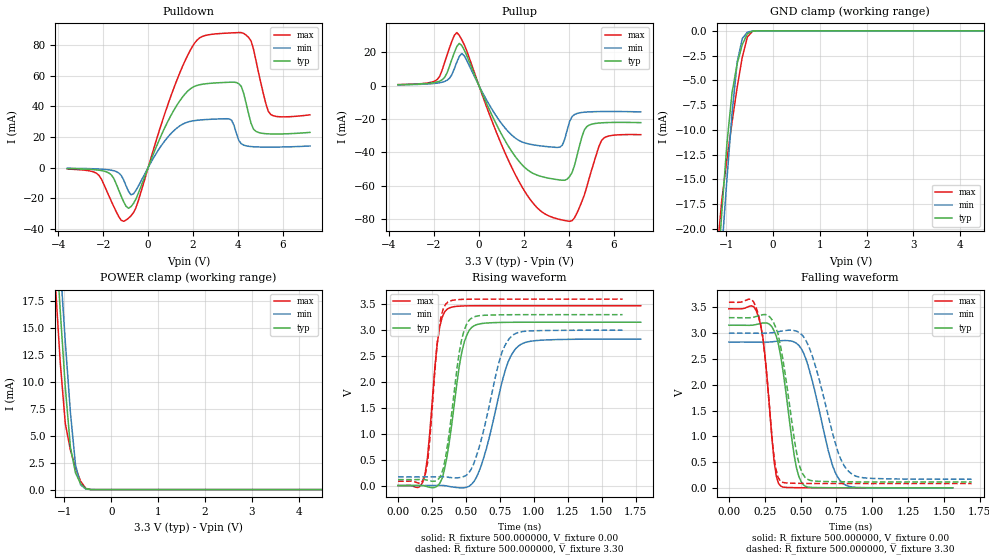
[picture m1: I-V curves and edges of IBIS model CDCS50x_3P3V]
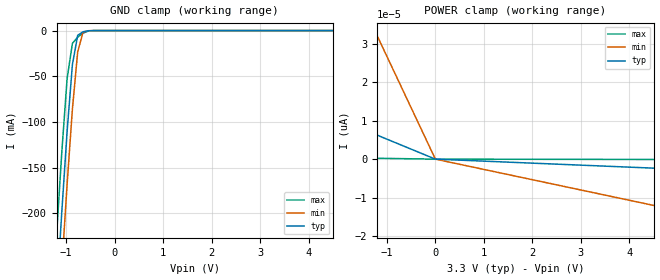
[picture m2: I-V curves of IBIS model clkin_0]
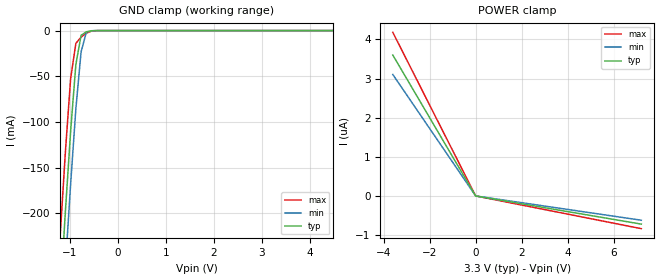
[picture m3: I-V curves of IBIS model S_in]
| TEXAS INSTRUMENTS INCORPORATED
| ASC / HSDC / CTS
| IBIS Model of CDCS504
| This file contains package information for the following:
| TSSOP-PW-8 package as [Component] CDCS504
| This device can be powered at the following Vccs:
| 3.3 volt
[IBIS Ver]   4.1
[Comment char]  |_char
[File Name]   cdcs504-q1.ibs
[File Rev]   1.0 | Simulation results only, no lab measurements
[Date]   April 27, 2017
[Source]   Model built from spectre simulations at:
   Texas Instruments Incorporated.
   Analog-eLab, HPA
   12500 TI Blvd
   Dallas, TX -75243
   For Support e-mail: webench_ibis_modeling@list.ti.com
[Notes]   Revision History
   Rev 1.0: 04/27/2017
[Disclaimer]  This model is designed as an aid for customers of Texas Instruments
 TI and its licensors and suppliers make no warranties, either expressed
 or implied, with respect to this  model, including the warranties of
 merchantability or fitness for a particular purpose.
 The model is provided solely on an "as is" basis. The entire risk as to
 its quality and performance is with the customer.
[Copyright] (C)Copyright 2017 Texas Instruments Incorporated.
   All rights reserved.
| Component TSSOP-PW-8 CDCS504
[Component]   CDCS504
[Manufacturer]   Texas Instruments, Inc.
[Package]
|   typ   min   max
R_pkg   0.747650e-01   0.368800e-01   1.126500e-01
L_pkg   1.018090e-09   0.602690e-09   1.433490e-09
C_pkg   1.006650e-13   6.656000e-14   1.347700e-13
[PIN]   signal_name   model_name   R_pin   L_pin   C_pin
1   IN   clkin_0   0.10191   1.26699e-09   0.08538e-12
2   GND   GND   0.10409   1.29915e-09   0.09128e-12
3   GND   POWER   0.05513   1.03439e-09   0.13141e-12
4   GND   POWER   0.08703   1.05334e-09   0.08277e-12
5   FS   S_in   0.03787   0.62719e-09   0.09930e-12
6   OUT   CDCS50x_3P3V   0.03688   0.60269e-09   0.09486e-12
7   OE   S_in   0.07828   0.93283e-09   0.06792e-12
8   VDD   POWER   0.07909   0.94459e-09   0.06676e-12
| Models and submodels in the file (3): CDCS50x_3P3V (Output), clkin_0 (Input), S_in (Input)
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[Model] CDCS50x_3P3V
|   Testbench Schematic CDCE949_3P3V model: Output
Model_type Output
Vmeas  =   1.50V
Cref   =   10.00pF
Rref   =   0
Vref   =   1.50V
| Variable   Typ   Min   Max
C_comp   1.113321e-12   1.105415e-12   1.124148e-12
[Temperature range]   27   105   -40
[Voltage range]   3.3   3.0   3.6
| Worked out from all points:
|   slope of the pulldown table from 0 to 0.495 V, typ, clamps not added: 27.4 ohm
|   slope of the pullup table from 0 to 0.495 V, typ, clamps not added: 32.4 ohm
|   GND clamp passes 1 mA (typ) near -0.62 V on its own axis
|   POWER clamp passes 1 mA (typ) near -0.70 V on its own axis
|   rising waveform, R_fixture 500.000000, V_fixture 0.00: 20-80 % time 101ps typ, 160ps min, 68.7ps max; typ from 0 V to 3.15 V
|   rising waveform, R_fixture 500.000000, V_fixture 3.30: 20-80 % time 94.9ps typ, 153ps min, 64.8ps max; typ from 0.114 V to 3.3 V
|   falling waveform, R_fixture 500.000000, V_fixture 0.00: 20-80 % time 92.3ps typ, 145ps min, 66.5ps max; typ from 3.15 V to 0 V
|   falling waveform, R_fixture 500.000000, V_fixture 3.30: 20-80 % time 102ps typ, 161ps min, 70.2ps max; typ from 3.3 V to 0.114 V
[GND Clamp]
|   Voltage   I(typ)   I(min)   I(max)
-3.6V     -211.8mA   -206.8mA   -215mA
-1.2V     -25.88mA   -29.69mA   -22.67mA
-1.091V   -18.26mA   -22.17mA   -17.07mA
-981.8mV  -11.37mA   -14.94mA   -12.96mA
-872.7mV  -6.231mA   -8.312mA   -9.209mA
-763.6mV  -3.327mA   -3.153mA   -5.704mA
-654.5mV  -1.39mA    -781.1uA   -2.657mA
-545.5mV  -297.7uA   -133.9uA   -616.4uA
-436.4mV  -24.67uA   -13.06uA   -40.52uA
-327.3mV  -1.017uA   -847.6nA   -796.5nA
7.2V      14.39pA    67.18pA    1.512pA
[POWER Clamp]
|   Voltage   I(typ)   I(min)   I(max)
-3.6V     210.6mA    205.6mA    214mA
-1.2V     24.42mA    28.43mA    19.54mA
-1.091V   16.68mA    20.92mA    11.88mA
-981.8mV  9.505mA    13.72mA    6.142mA
-872.7mV  3.945mA    7.17mA     3.66mA
-763.6mV  1.549mA    2.287mA    2.016mA
-654.5mV  547.6uA    435.9uA    771.4uA
-545.5mV  87.27uA    58.39uA    119.1uA
-436.4mV  5.106uA    4.537uA    4.472uA
-327.3mV  163.8nA    245.9nA    57.29nA
7.2V      -402.7pA   -2.184nA   -16.41pA
[Pulldown]
|   Voltage   I(typ)   I(min)   I(max)
-3.6V     -631.8uA   -409.9uA   -939.5uA
-2.291V   -1.486mA   -827.5uA   -3.72mA
-1.745V   -3.474mA   -1.437mA   -18.37mA
-763.6mV  -25.43mA   -17.7mA    -31.41mA
1.2V      38.75mA    24.8mA     54.02mA
2.618V    54.72mA    31.36mA    86.35mA
3.709V    55.67mA    30.96mA    87.77mA
4.036V    54.64mA    17.68mA    87.98mA
4.364V    41.7mA     14.19mA    86.27mA
4.691V    25.06mA    13.6mA     76.99mA
5.455V    21.95mA    13.36mA    34.63mA
7.2V      22.97mA    14.11mA    34.4mA
[Pullup]
|   Voltage   I(typ)   I(min)   I(max)
-3.6V     569.9uA    477.3uA    610.7uA
-1.855V   2.204mA    1.496mA    3.684mA
-981.8mV  23.45mA    14.14mA    31.77mA
-654.5mV  21.3mA     17.9mA     24.51mA
763.6mV   -22.86mA   -18.09mA   -27.52mA
1.855V    -46.48mA   -33.35mA   -59.2mA
2.727V    -54.22mA   -36.07mA   -74.83mA
3.709V    -56.66mA   -35.66mA   -80.48mA
4.364V    -41.87mA   -16.67mA   -76.22mA
4.8V      -24.54mA   -15.8mA    -60.5mA
5.455V    -22.28mA   -15.53mA   -32.88mA
7.2V      -22.17mA   -15.72mA   -29.37mA
[Ramp]
|  Variable  typ   min   max
dV/dt_r   1.946/1.041428e-10   1.741/1.650908e-10   2.143/7.067869e-11
dV/dt_f   1.946/1.041428e-10   1.741/1.650908e-10   2.143/7.067869e-11
R_load = 500.000000
[Rising waveform]
R_fixture = 500.000000
C_fixture = 0
L_fixture = 0
V_fixture = 0.00
V_fixture_min = 0.00
V_fixture_max = 0.00
|   Time   V(typ)   V(min)   V(max)
0s        8.739uV    -1.417uV   -47.05uV
198.6ps   -8.519mV   -152.9uV   210mV
288.9ps   -10.61mV   2.379mV    2.746V
361.2ps   571.7mV    -9.355mV   3.405V
469.5ps   2.577V     -44.41mV   3.467V
559.8ps   3.086V     80.06mV    3.472V
650.1ps   3.139V     707.2mV    3.473V
794.6ps   3.152V     2.267V     3.473V
884.9ps   3.154V     2.688V     3.473V
1.788ns   3.154V     2.828V     3.473V
[Rising waveform]
R_fixture = 500.000000
C_fixture = 0
L_fixture = 0
V_fixture = 3.30
V_fixture_min = 3.00
V_fixture_max = 3.60
|   Time   V(typ)   V(min)   V(max)
0s        114.5mV    167.2mV    83.33mV
200.5ps   113.4mV    167mV      214.5mV
233.9ps   90.53mV    167.2mV    884.2mV
300.8ps   132.8mV    169.3mV    3.032V
367.6ps   840.3mV    161.9mV    3.544V
451.2ps   2.578V     152.7mV    3.592V
534.7ps   3.221V     297mV      3.599V
751.9ps   3.297V     2.462V     3.6V
835.5ps   3.299V     2.882V     3.6V
1.654ns   3.3V       3V         3.6V
[Falling waveform]
R_fixture = 500.000000
C_fixture = 0
L_fixture = 0
V_fixture = 0.00
V_fixture_min = 0.00
V_fixture_max = 0.00
|   Time   V(typ)   V(min)   V(max)
0s        3.154V     2.828V     3.473V
204.8ps   3.178V     2.827V     3.332V
252.1ps   3.2V       2.826V     2.555V
315.1ps   3.044V     2.837V     518.5mV
362.4ps   2.535V     2.853V     31.86mV
456.9ps   601mV      2.828V     4.299mV
520ps     56.76mV    2.62V      2.085mV
709.1ps   2.462mV    559.9mV    240.3uV
787.8ps   1.214mV    106.8mV    91.56uV
1.56ns    -8.238uV   37.9uV     -1.099uV
[Falling waveform]
R_fixture = 500.000000
C_fixture = 0
L_fixture = 0
V_fixture = 3.30
V_fixture_min = 3.00
V_fixture_max = 3.60
|   Time   V(typ)   V(min)   V(max)
0s        3.3V       3V         3.6V
205.1ps   3.337V     2.999V     3.367V
239.3ps   3.36V      2.998V     2.857V
324.8ps   3.122V     3.02V      404.2mV
359ps     2.765V     3.037V     132.6mV
478.6ps   585.4mV    3.031V     87.91mV
547ps     167.6mV    2.801V     85.39mV
752.1ps   118.6mV    773.1mV    83.51mV
837.6ps   116.3mV    312.5mV    83.38mV
1.692ns   114.5mV    167.2mV    83.32mV
[Model] clkin_0
|   Testbench Schematic clkin_0 model: Input
Model_type Input
Vinl = 0.99   |--- Check this against the spec.
Vinh = 2.31   |--- Check this against the spec.
| Variable   Typ   Min   Max
C_comp   1.503583e-12   1.481523e-12   1.534573e-12
[Temperature range]   27   105   -40
[Voltage range]   3.300000   3.000000   3.600000
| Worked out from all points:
|   GND clamp passes 1 mA (typ) near -0.62 V on its own axis
[GND Clamp]
|   Voltage   I(typ)   I(min)   I(max)
-3.6V     -2.6A      -2.655A    -2.542A
-1.2V     -292mA     -353.4mA   -224.9mA
-1.091V   -198.3mA   -258.8mA   -132.9mA
-981.8mV  -110.4mA   -168.4mA   -52.65mA
-872.7mV  -37.24mA   -85.86mA   -14.03mA
-763.6mV  -5.214mA   -23.3mA    -7.194mA
-654.5mV  -1.311mA   -1.997mA   -2.858mA
-545.5mV  -241uA     -153.4uA   -518.3uA
-436.4mV  -18.85uA   -11.86uA   -29.59uA
7.2V      6.806pA    40.53pA    249.3fA
[POWER Clamp]
|   Voltage   I(typ)   I(min)   I(max)
-3.6V     21.84pA    107.8pA    748.4fA
-3.164V   17.86pA    88.92pA    624.2fA
-2.618V   13.85pA    70.2pA     495.1fA
-2.291V   11.91pA    61.2pA     430.7fA
-1.309V   6.805pA    34.97pA    246.1fA
-1.2V     6.238pA    32.06pA    225.6fA
0V        0A         0A         0A
7.2V      -3.743pA   -19.24pA   -135.4fA
[Model] S_in
|   Testbench Schematic S_in model: Input
Model_type Input
Vinl = 0.99   |--- Check this against the spec.
Vinh = 2.31   |--- Check this against the spec.
| Variable   Typ   Min   Max
C_comp   1.264527e-12   1.254747e-12   1.276839e-12
[Temperature range]   27   105   -40
[Voltage range]   3.300000   3.000000   3.600000
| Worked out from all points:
|   GND clamp passes 1 mA (typ) near -0.62 V on its own axis
[GND Clamp]
|   Voltage   I(typ)   I(min)   I(max)
-3.6V     -2.6A      -2.655A    -2.542A
-1.2V     -292mA     -353.4mA   -224.9mA
-1.091V   -198.3mA   -258.8mA   -132.9mA
-981.8mV  -110.4mA   -168.4mA   -52.65mA
-872.7mV  -37.24mA   -85.86mA   -14.03mA
-763.6mV  -5.216mA   -23.3mA    -7.197mA
-654.5mV  -1.314mA   -1.999mA   -2.86mA
-545.5mV  -244.2uA   -156.3uA   -521.9uA
-436.4mV  -22.51uA   -14.79uA   -34.11uA
7.2V      3.899uA    3.619uA    4.179uA
[POWER Clamp]
|   Voltage   I(typ)   I(min)   I(max)
-3.6V     3.599uA    3.102uA    4.179uA
-2.945V   2.945uA    2.538uA    3.419uA
0V        0A         0A         0A
7.2V      -719.8nA   -620.5nA   -835.8nA
